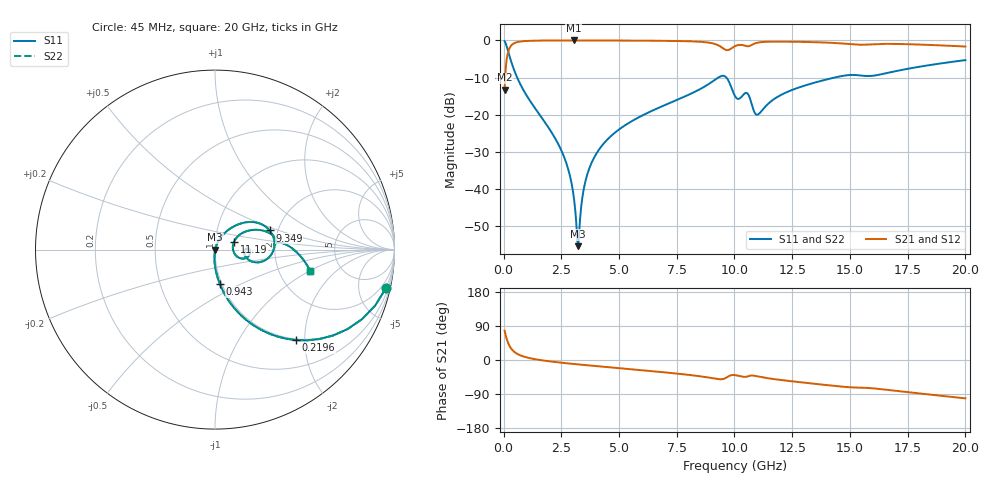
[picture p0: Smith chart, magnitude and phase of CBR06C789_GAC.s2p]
! S-parameter model data by Modelithics Inc.  support@modelithics.com 813-866-6335  Tampa FL USA
! S-Parameter data specifications:
! Substrate: 20-mil Rogers 4350B, substrate thickness, H=0.508mm, Dielectric constant, Er=3.75
! PCB Mounting Pad Footprint: Pad width, PadW=0.85mm , Pad length, PadL=0.64mm , Pad gap, PadG (edge-to-edge)=0.62mm , Reference planes=1.9mm apart
#  GHz  S  MA  R 50
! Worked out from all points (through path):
!   801 points, 45 MHz to 20 GHz, reference 50 ohm
!   highest |S21| = -0.02 dB at 3.038 GHz (marker M1); lowest = -13.3 dB at 45 MHz (marker M2)
!   group delay of S21, straight-line fit = 15.2 ps
!   lowest |S11| = -55.4 dB at 3.213 GHz (marker M3), VSWR 1.00, Z = 50.2 - j0.0763 ohm
!   |S11| at or under -10 dB: 589.4 MHz to 9.3 GHz (8.711 GHz wide, 176 % of centre); 9.651 GHz to 14.33 GHz (4.68 GHz wide, 39 % of centre)
!   |S22| runs from -55.4 to -0.2 dB; largest |S21 - S12| = 0
!   S11 on the Smith chart (normalised r, x): 45 MHz: 0.98, -8.91; 219.6 MHz: 0.98, -1.82; 943 MHz: 0.98, -0.39; 9.349 GHz: 1.81, +0.43; 11.19 GHz: 1.23, +0.11; 20 GHz: 3.00, -1.00
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0.045  0.9763 -12.7  0.2163 77.3  0.2163 77.3  0.9763 -12.7
0.219606  0.6771 -48.1  0.7354 41.8  0.7354 41.8  0.6771 -48.1
0.469044  0.3903 -68.6  0.92 21.3  0.92 21.3  0.3903 -68.6
0.942975  0.1937 -81.9  0.9801 7.8  0.9801 7.8  0.1937 -81.9
2.489488  0.03374 -94.6  0.9979 -7.0  0.9979 -7.0  0.03374 -94.6
2.8387  0.01665 -93.9  0.9982 -9.3  0.9982 -9.3  0.01665 -93.9
3.03825  0.007907 -88.8  0.9982 -10.5  0.9982 -10.5  0.007907 -88.8
3.212856  0.001704 -26.5  0.9982 -11.5  0.9982 -11.5  0.001704 -26.5
3.287688  0.003077 45.3  0.9982 -12.0  0.9982 -12.0  0.003077 45.3
3.387462  0.006755 62.9  0.9981 -12.5  0.9981 -12.5  0.006755 62.9
3.686787  0.018 70.1  0.9979 -14.3  0.9979 -14.3  0.018 70.1
4.260494  0.03836 69.6  0.9971 -17.5  0.9971 -17.5  0.03836 69.6
6.704981  0.1235 57.3  0.9885 -31.0  0.9885 -31.0  0.1235 57.3
9.349019  0.3227 19.3  0.8424 -50.8  0.8424 -50.8  0.3227 19.3
9.648344  0.317 -4.3  0.7416 -46.5  0.7416 -46.5  0.317 -4.3
10.0225  0.1783 -14.1  0.8359 -39.9  0.8359 -39.9  0.1783 -14.1
10.52138  0.1963 -6.2  0.8373 -44.1  0.8373 -44.1  0.1963 -6.2
10.92047  0.1016 -2.9  0.9187 -42.2  0.9187 -42.2  0.1016 -2.9
11.19486  0.1144 22.2  0.9505 -45.5  0.9505 -45.5  0.1144 22.2
13.36496  0.2645 24.5  0.9483 -62.1  0.9483 -62.1  0.2645 24.5
16.68248  0.3684 5.9  0.8983 -79.3  0.8983 -79.3  0.3684 5.9
20  0.5428 -12.5  0.8265 -101.2  0.8265 -101.2  0.5428 -12.5
